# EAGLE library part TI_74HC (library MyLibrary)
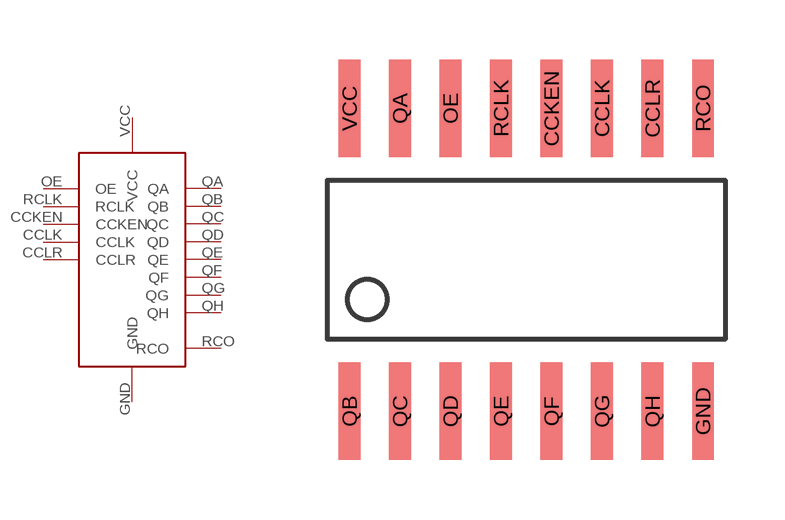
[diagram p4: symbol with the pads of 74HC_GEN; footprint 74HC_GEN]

Designator prefix -

## TI_74HC  [74HC_GEN]
CCKEN  CCKEN
CCLK  CCLK
CCLR  CCLR
GND  GND
OE  OE
QA  QA
QB  QB
QC  QC
QD  QD
QE  QE
QF  QF
QG  QG
QH  QH
RCLK  RCLK
RCO  RCO
VCC  VCC

## Footprint 74HC_GEN (pad centres in mm)
smd 0.55 x 2.45: CCKEN 0.635,3.81; CCLK 1.905,3.81; CCLR 3.175,3.81; GND 4.445,-3.81; OE -1.905,3.81; QA -3.175,3.81; QB -4.445,-3.81; QC -3.175,-3.81; QD -1.905,-3.81; QE -0.635,-3.81; QF 0.635,-3.81; QG 1.905,-3.81; QH 3.175,-3.81; RCLK -0.635,3.81; RCO 4.445,3.81; VCC -4.445,3.81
